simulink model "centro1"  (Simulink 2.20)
settings: Solver=VariableStepDiscrete  StartTime=0.0  StopTime=40.0  RelTol=1e-3  AbsTol=1e-6
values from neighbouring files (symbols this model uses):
  a = input('Inserisci il dato da graficare [1=PIDNL 2=PD 3=PID]: ')    [grp.m]    (also in grp1.m = input('Inserisci il dato da graficare [1..3]'))
undefined symbols (not defined in the file or in its folder): b
libraries: Puma x3, simulink x3

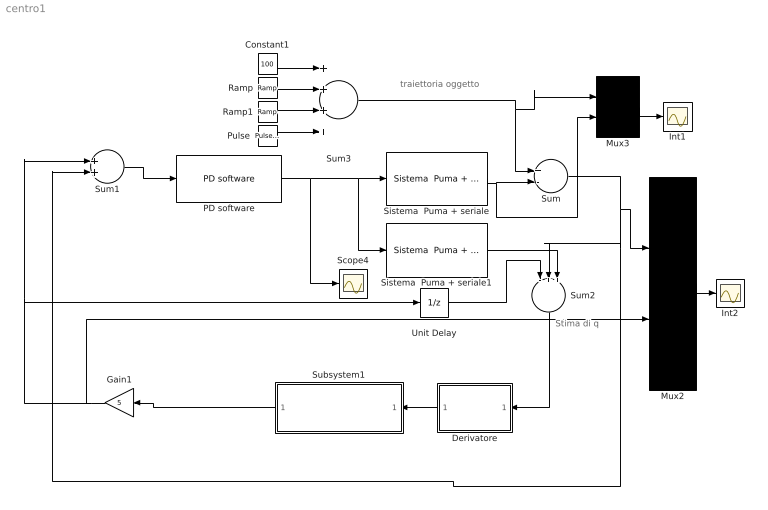
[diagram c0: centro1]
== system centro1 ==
  note: Stima di q
  note: traiettoria oggetto
  Constant1 : Constant  Value=100
  Derivatore : Subsystem  Orientation=left  mask(Simulazione Derivatore implementato in maniera software){Td=0.13, T=0.030, N=5}
      mask prompts: Td "Costante di derivazione Td"; T "Sample Time T del PD"; N "Indice polo del derivatore [5..10]"
      mask init:
      | Kbeta=Td/(N*T+Td);
      | Kalfa=N*Kbeta;
  Gain1 : Gain  Orientation=left  Gain=5
  Int1 : Scope
  Int2 : Scope
  Mux2 : Mux  Inputs=2
  Mux3 : Mux  Inputs=2
  PD software : Puma/PD software  Kp=0.5  Td=0.13  T=0.075  N=10
  "Pulse " : simulink/Sources/Pulse Generator  period=30  duty=10  amplitude=-50  start=30
  Ramp : simulink/Sources/Ramp  slope=-80  start=10  X0=0
  Ramp1 : simulink/Sources/Ramp  slope=+80  start=25  X0=0
  Scope4 : Scope
  Sistema  Puma + seriale : Puma/Sistema  Puma + seriale  Ts=.260
  Sistema  Puma + seriale1 : Puma/Sistema  Puma + seriale  Ts=.260
  Subsystem1 : Subsystem  Orientation=left  mask(Filtro di Butterworth){ordine=3, freq=0.1/16}
      mask prompts: ordine "Ordine del filtro"; freq "Parametro K per ricavare la Freq. di taglio Ft"
      mask help: Attenzione! Considerare il parametro Fc come la frequanza di campionamento del segnale di ingresso, per cui la frequanza di taglio diviene Ft=K*Fc;
      mask init:
      | [b,a]=butter(ordine,freq);
  Sum : Sum  Inputs=+-
  Sum1 : Sum  Inputs=++
  Sum2 : Sum  Orientation=down  Inputs=-++
  Sum3 : Sum  Inputs=++++
  Unit Delay : UnitDelay  X0=0  SampleTime=.320
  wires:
  Mux2/1 -> Int2/1
  Sistema  Puma + seriale/1 -> Sum/2, Mux3/2
  Sum2/1 -> Derivatore/1(In1)
  Constant1/1 -> Sum3/1
  Sum/1 -> Mux2/1, Sum2/2, Sum1/2
  Ramp/1 -> Sum3/2
  Ramp1/1 -> Sum3/3
  "Pulse "/1 -> Sum3/4
  Mux3/1 -> Int1/1
  Sum3/1 -> Sum/1, Mux3/1
  Derivatore/1(Out1) -> Subsystem1/1(In1)
  Gain1/1 -> Mux2/2, Sum1/1, Unit Delay/1
  Sum1/1 -> PD software/1
  PD software/1 -> Sistema  Puma + seriale/1, Sistema  Puma + seriale1/1, Scope4/1
  Subsystem1/1(Out1) -> Gain1/1
  Unit Delay/1 -> Sum2/1
  Sistema  Puma + seriale1/1 -> Sum2/3

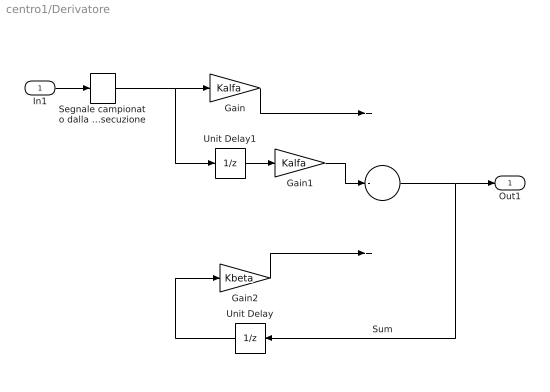
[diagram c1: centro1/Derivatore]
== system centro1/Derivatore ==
  In1 : Inport  Port=1  PortWidth=-1  SampleTime=-1
  Gain : Gain  Gain=Kalfa
  Gain1 : Gain  Gain=Kalfa
  Gain2 : Gain  Gain=Kbeta
  Segnale campionato dalla procedura software al momento del ciclo  d 'esecuzione : ZeroOrderHold  SampleTime=T
  Sum : Sum  Inputs=+-+
  Unit Delay : UnitDelay  Orientation=left  X0=0  SampleTime=T
  Unit Delay1 : UnitDelay  X0=0  SampleTime=T
  Out1 : Outport  Port=1
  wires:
  Gain1/1 -> Sum/2
  Unit Delay/1 -> Gain2/1
  Gain2/1 -> Sum/3
  Gain/1 -> Sum/1
  Unit Delay1/1 -> Gain1/1
  Sum/1 -> Out1/1, Unit Delay/1
  In1/1 -> Segnale campionato dalla procedura software al momento del ciclo  d 'esecuzione/1
  Segnale campionato dalla procedura software al momento del ciclo  d 'esecuzione/1 -> Gain/1, Unit Delay1/1

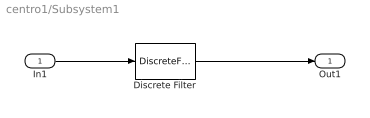
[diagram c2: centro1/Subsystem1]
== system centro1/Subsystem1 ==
  In1 : Inport  Port=1  PortWidth=-1  SampleTime=-1
  Discrete Filter : DiscreteFilter  Numerator=b  Denominator=a  SampleTime=.032
  Out1 : Outport  Port=1
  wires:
  In1/1 -> Discrete Filter/1
  Discrete Filter/1 -> Out1/1
